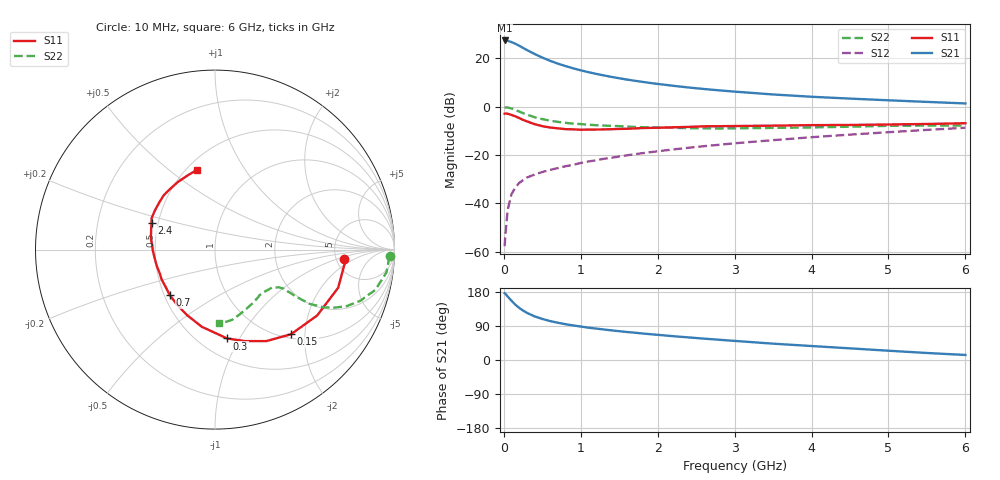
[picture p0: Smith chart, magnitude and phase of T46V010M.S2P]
! Infineon Technologies  Discrete & RF Semiconductors
! BFR182T
! Si NPN RF Bipolar Junction Transistor in SC75
! VCE = 6 V  IC = 10 mA
! Common Emitter S-Parameters:  October  1999
# GHz  S  MA  R  50
!  f  S11  S21  S12  S22
! GHz  MAG  ANG  MAG  ANG  MAG  ANG  MAG  ANG
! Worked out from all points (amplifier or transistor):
!   36 points, 10 MHz to 6 GHz, reference 50 ohm
!   highest |S21| = 27.5 dB at 10 MHz (marker M1)
!   |S21| within 3 dB of that: start of sweep to 245.1 MHz
!   unconditionally stable (mu >= 1): 1.094 GHz to 3.891 GHz
!   at 250 MHz: K = 0.43, MSG = 27.4 dB, |S12| = -30.4 dB
!   at 1.4 GHz: K = 1.06, MAG = 15.3 dB, |S12| = -21.1 dB
!   at 6 GHz: K = 0.86, MSG = 5.0 dB, |S12| = -8.7 dB
!   lowest NFmin = 1.50 dB at 450 MHz
!   S11 on the Smith chart (normalised r, x): 10 MHz: 5.80, -1.32; 150 MHz: 1.08, -1.70; 300 MHz: 0.67, -0.89; 700 MHz: 0.53, -0.31; 2.4 GHz: 0.46, +0.16; 6 GHz: 0.56, +0.63
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0.01  0.7186 -4.4  23.6 176.2  0.0013 84.1  0.9735 -2.2
0.02  0.7282 -5.4  23.5 175.0  0.0022 92.4  0.9711 -2.9
0.05  0.7184 -17.2  23.19 167.4  0.0074 87.0  0.9641 -7.5
0.1  0.6774 -32.8  21.83 156.3  0.0156 78.1  0.9213 -14.1
0.15  0.6338 -48.1  20.16 145.9  0.0213 69.7  0.8581 -19.4
0.2  0.5843 -60.8  18.34 137.5  0.0266 67.2  0.7976 -23.3
0.25  0.5358 -72.0  16.54 130.4  0.0302 63.0  0.738 -26.0
0.3  0.4997 -82.2  14.95 124.5  0.0343 60.7  0.6896 -27.9
0.4  0.4365 -99.6  12.37 115.0  0.0395 59.3  0.6085 -29.8
0.5  0.397 -113.1  10.44 108.3  0.0446 58.7  0.5553 -30.0
0.6  0.3722 -124.9  8.951 102.8  0.0493 59.5  0.5165 -30.1
0.7  0.3577 -134.7  7.855 98.4  0.0537 59.8  0.4867 -29.9
0.9  0.3408 -150.9  6.257 91.3  0.0628 62.1  0.4478 -29.8
1.1  0.3367 -163.4  5.205 85.3  0.0737 63.2  0.4259 -30.2
1.4  0.3433 -176.4  4.15 78.2  0.088 64.5  0.4026 -31.7
1.6  0.3505 175.8  3.657 73.9  0.0988 65.1  0.3889 -32.8
2.2  0.3754 161.3  2.72 62.9  0.1307 65.8  0.3667 -38.7
2.4  0.3828 157.5  2.508 59.6  0.1416 65.7  0.3603 -41.1
3.5  0.4066 139.9  1.798 43.1  0.2038 62.9  0.3652 -55.1
4.5  0.4202 126.7  1.476 30.7  0.265 58.6  0.3868 -69.5
5.5  0.4402 110.4  1.261 18.5  0.3324 53.4  0.4076 -81.8
6  0.4563 102.5  1.172 13.3  0.3676 49.9  0.4084 -86.8
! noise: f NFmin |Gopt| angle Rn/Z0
0.45  1.5  0.26  43  0.28
0.9  1.6  0.24  87  0.22
1.8  2.1  0.2  170  0.2
